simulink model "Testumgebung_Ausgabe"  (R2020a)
settings: Solver=ode4  StartTime=0.0  StopTime=Simulationszeit  FixedStep=0.01  RelTol=1e-3
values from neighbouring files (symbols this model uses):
  Gierrate_value = (b-a).*rand(1,1) + a    [Testskript_Ausgabe.m]    (also in Single_TestSkript_Hinterachse.m = 2; Testskript_Hinterachse.m; Single_Testskript_Karosserie.m = 2; Testskript_Karosserie.m)
  Kraeftesumme_X_value = (b-a).*rand(1,1) + a    [Testskript_Ausgabe.m]
  Kraeftesumme_Y_value = (b-a).*rand(1,1) + a    [Testskript_Ausgabe.m]
  Langsgeschwindigkeit_value = (b-a).*rand(1,1) + a    [Testskript_Ausgabe.m]
  Querbeschleunigung_value = (b-a).*rand(1,1) + a    [Testskript_Ausgabe.m]    (also in Single_Testskript_Karosserie.m = 3; Testskript_Karosserie.m)
  Schwimmwinkel_value = (b-a).*rand(1,1) + a    [Testskript_Ausgabe.m]    (also in Single_TestSkript_Hinterachse.m = 1.3; Testskript_Hinterachse.m; Single_Testskript_Vorderachse.m = 1.3; Testskript_Vorderachse.m)

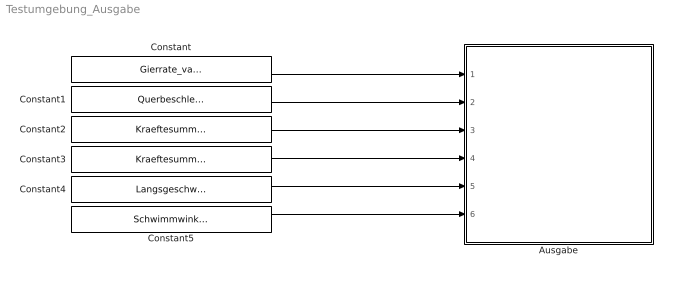
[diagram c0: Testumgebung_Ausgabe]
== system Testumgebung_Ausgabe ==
  Ausgabe : Subsystem
  Constant : Constant  Value=Gierrate_value
  Constant1 : Constant  Value=Querbeschleunigung_value
  Constant2 : Constant  Value=Kraeftesumme_X_value
  Constant3 : Constant  Value=Kraeftesumme_Y_value
  Constant4 : Constant  Value=Langsgeschwindigkeit_value
  Constant5 : Constant  Value=Schwimmwinkel_value
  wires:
  Constant/1 -> Ausgabe/1(Gierrate K_psi_punkt)
  Constant1/1 -> Ausgabe/2(Querbeschleunigung KaCy)
  Constant2/1 -> Ausgabe/3(Summenkraft KFcx)
  Constant3/1 -> Ausgabe/4(Summenkraft KFcy)
  Constant4/1 -> Ausgabe/5(Fahrzeuglängsgeschwindigkeit KvCx)
  Constant5/1 -> Ausgabe/6(Schwimmwinkel beta)

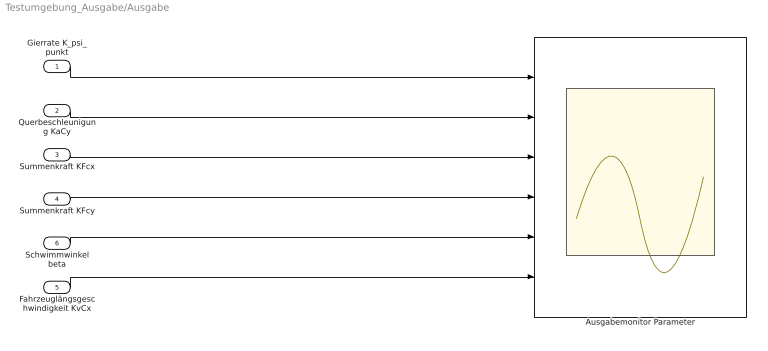
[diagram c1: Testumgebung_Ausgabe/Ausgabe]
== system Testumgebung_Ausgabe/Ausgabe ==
  Gierrate K_psi_punkt : Inport
  Querbeschleunigung KaCy : Inport  Port=2
  Summenkraft KFcx : Inport  Port=3
  Summenkraft KFcy : Inport  Port=4
  Fahrzeuglängsgeschwindigkeit KvCx : Inport  Port=5
  Schwimmwinkel beta : Inport  Port=6
  Ausgabemonitor Parameter : Scope  NumInputPorts=6
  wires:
  Gierrate K_psi_punkt/1 -> Ausgabemonitor Parameter/1
  Querbeschleunigung KaCy/1 -> Ausgabemonitor Parameter/2
  Summenkraft KFcx/1 -> Ausgabemonitor Parameter/3
  Summenkraft KFcy/1 -> Ausgabemonitor Parameter/4
  Schwimmwinkel beta/1 -> Ausgabemonitor Parameter/5
  Fahrzeuglängsgeschwindigkeit KvCx/1 -> Ausgabemonitor Parameter/6
